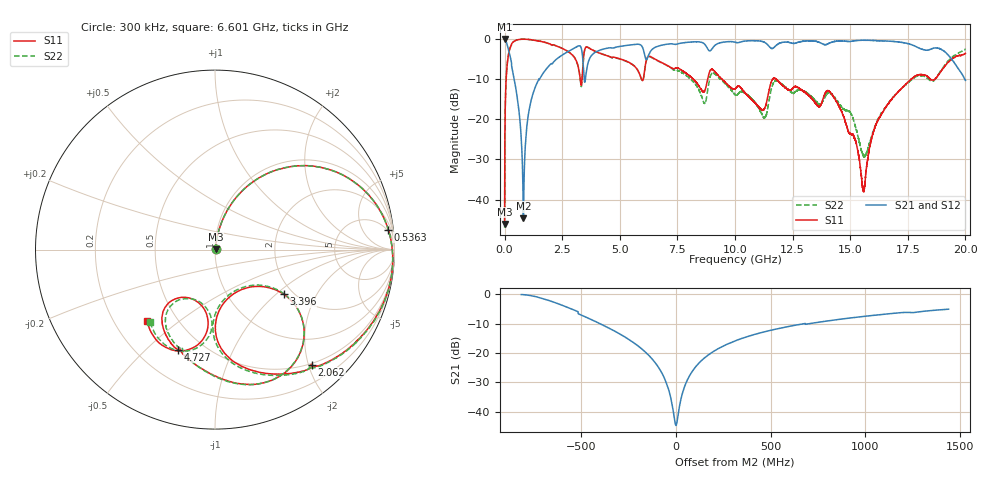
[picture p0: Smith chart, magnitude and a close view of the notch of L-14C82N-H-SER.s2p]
!{L-14C82N}
!Johanson Technology Inc.
!www.johansontechnology.com
!Test Board Conditions:
!Substrate Type  RO4350B
!Substrate Thickness  20 mil
!Substrate Dk  3.66
!TL Type: GCPW
!TL Trace Width  36 mil
!TL Gap  12 mil
!Electrode orientation  Horizontal
!DUT TOPOLOGY	SERIES
!Mounting Pad LxW  26x36 mil
! Created Sun Jun 20 13:08:27 2021
# hz S ma R 50
! 2 Port Network Data from SP1.SP block
! freq  magS11  angS11  magS21  angS21  magS12  angS12  magS22  angS22
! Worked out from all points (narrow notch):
!   20001 points, 300 kHz to 20 GHz, reference 50 ohm
!   highest |S21| = -0.03 dB at 1.3 MHz (marker M1); lowest = -44.7 dB at 816.3 MHz (marker M2)
!   notch at M2: 43.3 dB deep, 240 MHz wide at half that depth
!   lowest |S11| = -46.0 dB at 300 kHz (marker M3), VSWR 1.01, Z = 50.5 + j0.135 ohm
!   |S11| at or under -10 dB: 8.191 GHz to 8.814 GHz (623.6 MHz wide, 7.33 % of centre); 9.43 GHz to 11.63 GHz (2.202 GHz wide, 20.9 % of centre); 11.8 GHz to 17.64 GHz (5.845 GHz wide, 39.7 % of centre)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
!   |S22| runs from -47.0 to 0.0 dB; largest |S21 - S12| = 0.013
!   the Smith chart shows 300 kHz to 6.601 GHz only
!   S11 on the Smith chart (normalised r, x): 300 kHz: 1.01, +0.00; 536.3 MHz: 4, +16; 2.062 GHz: 0.47, -2.06; 3.396 GHz: 1.79, -1.12; 4.727 GHz: 0.37, -0.63; 6.601 GHz: 0.34, -0.38
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300000  0.004991 15.5  0.9955 -0.2  0.9954 -0.2  0.004482 19.0
1300000  0.007115 64.7  0.9969 -0.4  0.9968 -0.5  0.007275 63.9
1.433e8  0.5746 51.3  0.7943 -36.6  0.7955 -36.5  0.5764 51.1
5.363e8  0.9718 6.6  0.1974 -81.2  0.1975 -81.1  0.9725 6.4
8.163e8  0.9945 -7.3  0.005827 -8.4  0.005844 -8.2  0.9936 -7.7
1.1983e9  0.9723 -22.4  0.193 65.7  0.1933 65.6  0.9748 -22.9
2.0623e9  0.839 -50.0  0.4898 36.5  0.4897 36.5  0.8345 -51.0
3.3343e9  0.2672 -57.1  0.7561 -32.3  0.7571 -32.3  0.2564 -58.3
3.3963e9  0.4567 -33.0  0.5531 -45.4  0.5533 -45.4  0.448 -32.6
3.6473e9  0.7768 -75.3  0.5319 6.8  0.5328 6.9  0.7774 -75.5
4.7273e9  0.5936 -110.3  0.7724 -22.2  0.7739 -22.3  0.5786 -108.2
6.6013e9  0.5473 -133.8  0.8016 -46.9  0.8045 -46.6  0.5406 -132.1
6.6673e9  0.5339 -135.7  0.8152 -48.4  0.8169 -48.2  0.5292 -134.2
1.00003e10  0.2392 -167.2  0.9119 -103.7  0.9133 -103.7  0.2038 172.4
1.12683e10  0.1349 -165.0  0.9115 -127.5  0.9133 -127.5  0.1053 177.4
1.17583e10  0.3188 170.0  0.8171 -122.7  0.8184 -122.7  0.2993 177.2
1.33343e10  0.1812 117.9  0.9437 -148.7  0.9433 -148.7  0.189 141.5
1.43873e10  0.1691 99.1  0.9361 -160.5  0.9364 -160.7  0.1766 142.8
1.55713e10  0.01307 164.1  0.9651 178.9  0.9639 178.8  0.03538 -178.7
1.66673e10  0.1572 -126.7  0.9398 158.3  0.936 158.3  0.1587 -123.8
1.89493e10  0.3995 -172.6  0.7435 114.6  0.7464 114.5  0.4107 171.0
2e10  0.6612 140.8  0.3041 105.2  0.2989 105.6  0.7439 120.6
